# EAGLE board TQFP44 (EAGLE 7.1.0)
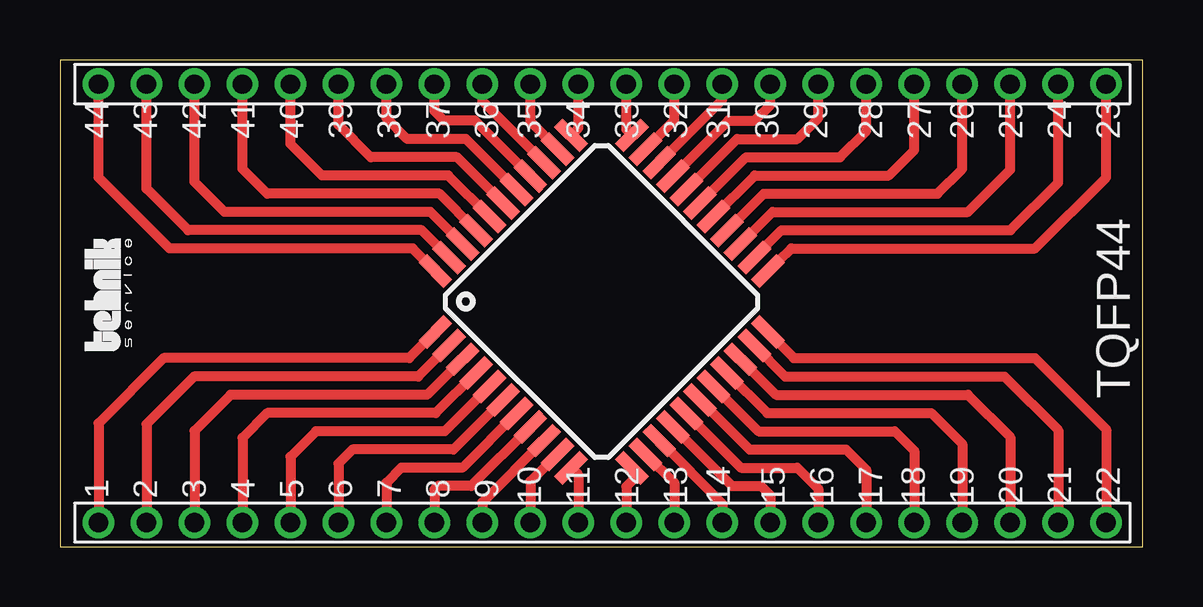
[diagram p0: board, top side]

Size 45.14 x 20.31 mm. Coordinates in mm from the lower left corner, seen from the top.
Outline: 0,0 45.14,0 45.14,20.31 0,20.31 0,0
Copper layers (1*16): Top 0.035mm / dielectric 1.5mm / Bottom 0.035mm
Design rules "default": minimum track width 10mil, minimum drill 24mil, track to track 8mil, track to pad 8mil, pad to pad 8mil, via to via 8mil, smd to smd 8mil, copper to edge 40mil, drill to drill 8mil, minimum pad ring 10mil, minimum via ring 8mil, stop-mask expansion 4mil, vias tented up to drill 0mil, thermal gap 10mil

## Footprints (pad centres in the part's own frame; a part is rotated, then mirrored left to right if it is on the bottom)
TQFP44 = smd 1.5 x 0.5: 1 -5.8,4; 2 -5.8,3.2; 3 -5.8,2.4; 4 -5.8,1.6; 5 -5.8,0.8; 6 -5.8,0; 7 -5.8,-0.8; 8 -5.8,-1.6; 9 -5.8,-2.4; 10 -5.8,-3.2; 11 -5.8,-4; 23 5.8,-4; 24 5.8,-3.2; 25 5.8,-2.4; 26 5.8,-1.6; 27 5.8,-0.8; 28 5.8,0; 29 5.8,0.8; 30 5.8,1.6; 31 5.8,2.4; 32 5.8,3.2; 33 5.8,4 | smd 0.5 x 1.5: 12 -4,-5.8; 13 -3.2,-5.8; 14 -2.4,-5.8; 15 -1.6,-5.8; 16 -0.8,-5.8; 17 0,-5.8; 18 0.8,-5.8; 19 1.6,-5.8; 20 2.4,-5.8; 21 3.2,-5.8; 22 4,-5.8; 34 4,5.8; 35 3.2,5.8; 36 2.4,5.8; 37 1.6,5.8; 38 0.8,5.8; 39 0,5.8; 40 -0.8,5.8; 41 -1.6,5.8; 42 -2.4,5.8; 43 -3.2,5.8; 44 -4,5.8
1X22 = drill 0.8: 1 -21,0; 2 -19,0; 3 -17,0; 4 -15,0; 5 -13,0; 6 -11,0; 7 -9,0; 8 -7,0; 9 -5,0; 10 -3,0; 11 -1,0; 12 1,0; 13 3,0; 14 5,0; 15 7,0; 16 9,0; 17 11,0; 18 13,0; 19 15,0; 20 17,0; 21 19,0; 22 21,0

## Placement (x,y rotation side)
1  [TQFP44]  22.58,10.23 45 top
2  1X22THM  [1X22]  22.61,1.02 0 top
U$1  [LOGOT]  3.05,8.13 90 top
U$3  1X22THM  [1X22]  22.61,19.3 180 top

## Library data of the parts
1 = atmel; MPN: ATMEGA32-16AU; OC_FARNELL: 9171274; OC_NEWARK: 69K6677
2 U$3 = adafruit
U$1 = logoo

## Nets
1: 1.1 2.1
2: 1.2 2.2
3: 1.3 2.3
4: 1.4 2.4
5: 1.5 2.5
6: 1.6 2.6
7: 1.7 2.7
8: 1.8 2.8
9: 1.9 2.9
10: 1.10 2.10
11: 1.11 2.11
12: 1.12 2.12
13: 1.13 2.13
14: 1.14 2.14
15: 1.15 2.15
16: 1.16 2.16
17: 1.17 2.17
18: 1.18 2.18
19: 1.19 2.19
20: 1.20 2.20
21: 1.21 2.21
22: 1.22 2.22
23: 1.23 U$3.1
24: 1.24 U$3.2
25: 1.25 U$3.3
26: 1.26 U$3.4
27: 1.27 U$3.5
28: 1.28 U$3.6
29: 1.29 U$3.7
30: 1.30 U$3.8
31: 1.31 U$3.9
32: 1.32 U$3.10
33: 1.33 U$3.11
34: 1.34 U$3.12
35: 1.35 U$3.13
36: 1.36 U$3.14
37: 1.37 U$3.15
38: 1.38 U$3.16
39: 1.39 U$3.17
40: 1.40 U$3.18
41: 1.41 U$3.19
42: 1.42 U$3.20
43: 1.43 U$3.21
44: 1.44 U$3.22

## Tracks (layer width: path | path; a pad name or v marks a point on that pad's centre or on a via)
1
  Top 0.406: 1.1 14.56,7.87 4.32,7.87 1.61,5.16 2.1
2
  Top 0.406: 1.2 14.93,7.11 5.59,7.11 3.61,5.13 2.2
3
  Top 0.406: 1.3 15.3,6.35 7.11,6.35 5.61,4.84 2.3
4
  Top 0.406: 1.4 15.67,5.59 8.64,5.59 7.61,4.56 2.4
5
  Top 0.406: 1.5 16.04,4.83 10.67,4.83 9.61,3.76 2.5
6
  Top 0.406: 1.6 16.4,4.06 12.19,4.06 11.61,3.48 2.6
7
  Top 0.406: 1.7 16.77,3.3 14.22,3.3 13.61,2.68 2.7
8
  Top 0.406: 1.8 17.14,2.54 15.75,2.54 15.61,2.4 2.8
9
  Top 0.406: 1.9 17.61,1.87 2.9
10
  Top 0.406: 1.10 19.61,2.74 2.10
11
  Top 0.406: 1.11 21.61,3 2.11
12
  Top 0.406: 1.12 23.88,3.28 23.88,2.79 23.61,2.52 2.12
13
  Top 0.406: 1.13 25.61,2.68 2.13
14
  Top 0.406: 1.14 27.61,1.81 2.14
15
  Top 0.406: 1.15 28.01,2.54 29.21,2.54 29.61,2.14 2.15
16
  Top 0.406: 1.16 28.38,3.3 30.73,3.3 31.61,2.43 2.16
17
  Top 0.406: 1.17 28.75,4.06 32.77,4.06 33.61,3.22 2.17
18
  Top 0.406: 1.18 29.11,4.83 34.8,4.83 35.61,4.02 2.18
19
  Top 0.406: 1.19 29.48,5.59 36.32,5.59 37.61,4.3 2.19
20
  Top 0.406: 1.20 29.85,6.35 37.85,6.35 39.61,4.59 2.20
21
  Top 0.406: 1.21 30.22,7.11 39.37,7.11 41.61,4.88 2.21
22
  Top 0.406: 1.22 30.59,7.87 40.64,7.87 43.61,4.91 2.22
23
  Top 0.406: 1.23 29.94,11.94 29.97,11.94 30.48,12.45 40.64,12.45 43.61,15.41 U$3.1
24
  Top 0.406: 1.24 30.07,13.21 39.62,13.21 41.61,15.19 U$3.2
25
  Top 0.406: 1.25 29.7,13.97 37.85,13.97 39.61,15.73 U$3.3
26
  Top 0.406: 1.26 29.34,14.73 36.58,14.73 37.61,15.76 U$3.4
27
  Top 0.406: 1.27 28.97,15.49 34.54,15.49 35.61,16.56 U$3.5
28
  Top 0.406: 1.28 28.6,16.26 32.51,16.26 33.61,17.35 U$3.6
29
  Top 0.406: 1.29 28.23,17.02 30.73,17.02 31.61,17.89 U$3.7
30
  Top 0.406: 1.30 27.86,17.78 28.96,17.78 29.61,18.43 U$3.8
31
  Top 0.406: 1.31 27.61,18.66 U$3.9
32
  Top 0.406: 1.32 25.61,17.79 U$3.10
33
  Top 0.406: 1.33 23.61,17.41 U$3.11
34
  Top 0.406: 1.34 21.61,17.47 U$3.12
35
  Top 0.406: 1.35 19.61,17.73 U$3.13
36
  Top 0.406: 1.36 17.61,18.6 U$3.14
37
  Top 0.406: 1.37 17.29,17.78 16,17.78 15.61,18.18 U$3.15
38
  Top 0.406: 1.38 16.92,17.02 14.48,17.02 13.61,17.89 U$3.16
39
  Top 0.406: 1.39 16.55,16.26 12.95,16.26 11.61,17.6 U$3.17
40
  Top 0.406: 1.40 16.18,15.49 10.92,15.49 9.61,16.81 U$3.18
41
  Top 0.406: 1.41 15.81,14.73 8.64,14.73 7.61,15.76 U$3.19
42
  Top 0.406: 1.42 15.45,13.97 6.86,13.97 5.61,15.22 U$3.20
43
  Top 0.406: 1.43 15.08,13.21 5.33,13.21 3.61,14.94 U$3.21
44
  Top 0.406: 1.44 14.71,12.45 4.57,12.45 1.61,15.41 U$3.22

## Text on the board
tNames: 44 | 43 | 42 | 41 | 40 | 39 | 38 | 37 | 36 | 35 | 34 | 33 | 32 | 31 | 30 | 29 | 28 | 27 | 26 | 25 | 24 | 23 | TQFP44 | 1 | 2 | 3 | 4 | 5 | 6 | 7 | 8 | 9 | 10 | 11 | 12 | 13 | 14 | 15 | 16 | 17 | 18 | 19 | 20 | 21 | 22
